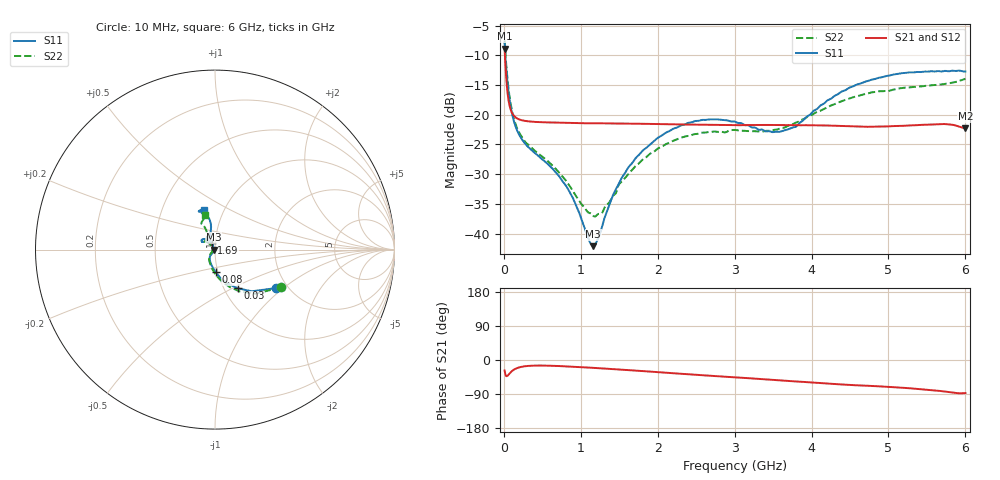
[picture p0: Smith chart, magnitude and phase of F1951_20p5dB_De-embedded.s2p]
! Integrated Device Technology
! Corporate Headquarters
! 6024 Silver Creek Valley Road
! San Jose, CA 95138  USA
! Phone:  1-408-284-8200
! Toll Free:  1-800-223-1366
! Webpage:  http://www.idt.com/
! Timing and RF Division
! 515 Groton Road, Suite 102
! Westford, MA 01886-6024
! Device:  F1951
! Description: 6-bit 0.5 dB Digital Step Attenuator
! Frequency:  100.0 -  4000.00 MHz
! Package:  4x4 mm Thin QFN Plastic Package: 24 pin
! Ports:  2 RF, 6 DC
!  Pin  1  = NC
!  Pin  2  = RF1  =  Port 1
!  Pin  3  = GND
!  Pin  4  = NC
!  Pin  5  = Serial Data Out (SDO)
!  Pin  6  = NC
!  Pin  7  = Reset Bar ( RSTb)
!  Pin  8  = Clock (CLK)
!  Pin  9  = Chip Select Bar (CSb)
!  Pin 10  = NC
!  Pin 11  = Serial Data In (SDI)
!  Pin 12  = NC
!  Pin 13  = NC
!  Pin 14  = VDD
!  Pin 15  = NC
!  Pin 16  = GND
!  Pin 17  = RF2  =  Port 2
!  Pin 18  = NC
!  Pin 19  = GND
!  Pin 20  = GND
!  Pin 21  = GND
!  Pin 22  = GND
!  Pin 23  = GND
!  Pin 24  = GND
! State:  41
! Atten State:  20.5 dB
! Voltage:  +3.30 Volts
! Current:  0.490 mA
! Data:  The device was measured on a F195X evaluation board which has
!  individual transmission lines to the RF pins.  Data was collected
!  de-embedded using a Automatic Fixture Removal [AFR] (Keysight Technologies).
!  The reference plane is the edge of the package pin.
! Misc:  Lot Code  1225BCA
!  Action Tracker AT0399
! Date Measured:  2018-09-13
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# GHz S dB R 50
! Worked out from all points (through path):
!   600 points, 10 MHz to 6 GHz, reference 50 ohm
!   highest |S21| = -8.86 dB at 10 MHz (marker M1); lowest = -22.3 dB at 6 GHz (marker M2)
!   group delay of S21, straight-line fit = 34.3 ps
!   lowest |S11| = -42.1 dB at 1.16 GHz (marker M3), VSWR 1.02, Z = 49.2 + j0.0536 ohm
!   |S11| at or under -10 dB: 19.24 MHz to end of sweep
!   |S22| runs from -37.1 to -7.5 dB; largest |S21 - S12| = 0.00023
!   S11 on the Smith chart (normalised r, x): 10 MHz: 1.74, -0.89; 30 MHz: 1.16, -0.53; 80 MHz: 0.98, -0.25; 1.69 GHz: 0.96, +0.07; 6 GHz: 0.80, +0.38
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0.01  -7.90 -32.1  -8.86 -27.7  -8.87 -27.7  -7.50 -30.0
0.03  -12.02 -59.5  -13.58 -42.5  -13.58 -42.5  -11.36 -59.5
0.05  -14.92 -74.3  -16.54 -41.2  -16.54 -41.2  -14.34 -75.4
0.08  -17.96 -88.2  -18.76 -34.3  -18.77 -34.3  -17.47 -89.9
0.15  -21.88 -106.9  -20.42 -23.3  -20.41 -23.3  -21.48 -108.5
0.25  -24.41 -119.5  -20.97 -17.3  -20.97 -17.2  -24.10 -122.1
0.72  -30.38 -126.8  -21.34 -16.0  -21.33 -16.0  -29.76 -136.3
0.88  -33.58 -128.8  -21.38 -17.6  -21.38 -17.6  -32.48 -140.8
1.01  -37.61 -137.4  -21.42 -19.0  -21.42 -19.0  -35.06 -149.2
1.16  -42.13 176.0  -21.44 -20.7  -21.44 -20.6  -36.97 -173.0
1.27  -39.15 133.1  -21.44 -22.0  -21.44 -22.0  -36.61 164.0
1.44  -32.96 117.2  -21.48 -24.3  -21.48 -24.3  -33.42 142.6
1.69  -27.74 116.5  -21.50 -27.6  -21.50 -27.7  -28.94 132.4
2.01  -23.82 125.1  -21.57 -32.2  -21.57 -32.2  -25.62 134.9
2.49  -21.05 138.6  -21.66 -38.9  -21.66 -38.9  -23.25 142.5
3.01  -21.19 148.8  -21.75 -45.9  -21.75 -45.9  -22.56 146.2
3.58  -22.89 128.0  -21.73 -53.6  -21.73 -53.6  -22.34 129.0
3.79  -22.05 112.1  -21.78 -56.5  -21.78 -56.5  -21.36 122.0
4.01  -19.57 102.9  -21.77 -59.5  -21.77 -59.5  -19.99 116.5
4.49  -15.46 100.1  -21.95 -65.7  -21.94 -65.7  -17.28 114.7
5.01  -13.41 108.3  -21.95 -70.9  -21.95 -70.9  -15.97 117.3
6  -12.72 105.5  -22.26 -87.2  -22.26 -87.2  -13.94 106.4
